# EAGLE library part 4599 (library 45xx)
8-bit addressable LATCH
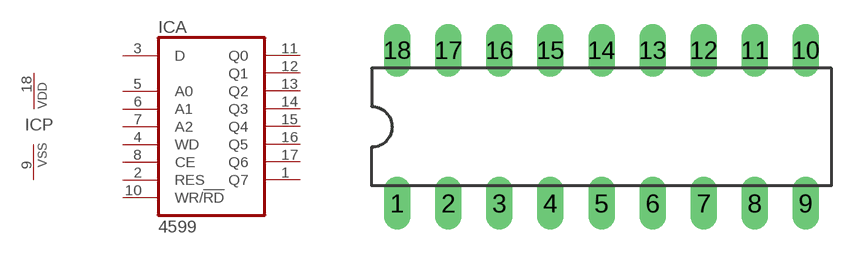
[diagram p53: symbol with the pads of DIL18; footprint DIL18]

Designator prefix IC; gates A=4599 P=PWRN

## 4599N  [DIL18]
1  A:Q7  out
2  A:RES  in
3  A:D
4  A:WD  in
5  A:A0  in
6  A:A1  in
7  A:A2  in
8  A:CE  in
9  P:VSS  pwr
10  A:WR/!RD  in
11  A:Q0  out
12  A:Q1  out
13  A:Q2  out
14  A:Q3  out
15  A:Q4  out
16  A:Q5  out
17  A:Q6  out
18  P:VDD  pwr

## Footprint DIL18 (pad centres in mm)
Dual In Line Package
drill 0.813 long: 1 -10.16,-3.81; 2 -7.62,-3.81; 3 -5.08,-3.81; 4 -2.54,-3.81; 5 0,-3.81; 6 2.54,-3.81; 7 5.08,-3.81; 8 7.62,-3.81; 9 10.16,-3.81; 10 10.16,3.81; 11 7.62,3.81; 12 5.08,3.81; 13 2.54,3.81; 14 0,3.81; 15 -2.54,3.81; 16 -5.08,3.81; 17 -7.62,3.81; 18 -10.16,3.81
